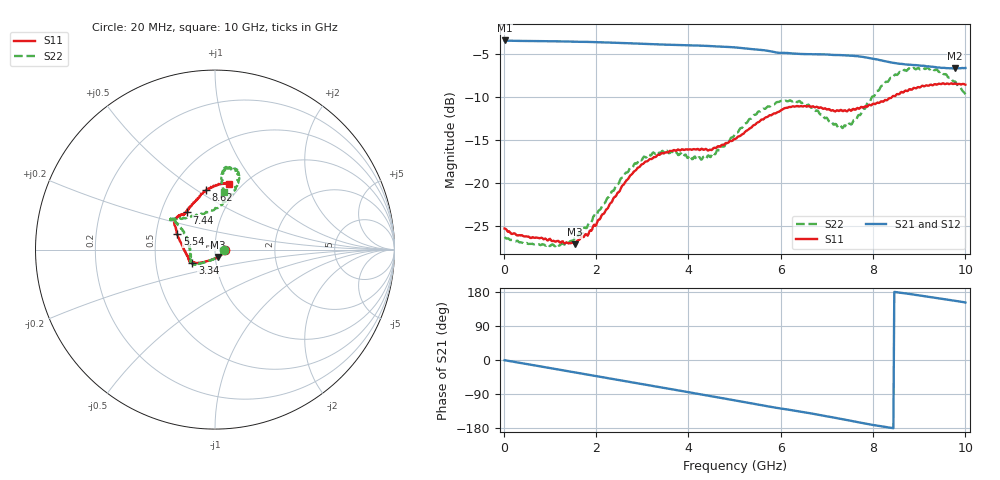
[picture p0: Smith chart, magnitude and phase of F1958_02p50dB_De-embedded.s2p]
! Integrated Device Technology
! Corporate Headquarters
! 6024 Silver Creek Valley Road
! San Jose, CA 95138  USA
! Phone:  1-408-284-8200
! Toll Free:  1-800-223-1366
! Webpage:  http://www.idt.com/
! Timing and RF Division
! 515 Groton Road, Suite 102
! Westford, MA 01886-6024
! Device:  F1958
! Description: 7-bit 0.25 dB Digital Step Attenuator
! Frequency:  0.001 -  6.000 GHz
! Package:  4x4 mm Thin QFN Plastic Package: 24 pin
! Ports:  2 RF, 12 DC
!  Pin  1  = D0
!  Pin  2  = VDD
!  Pin  3  = VMODE
!  Pin  4  = GND
!  Pin  5  = RF1  =  Port 1
!  Pin  6  = GND
!  Pin  7  = GND
!  Pin  8  = GND
!  Pin  9  = GND
!  Pin 10  = GND
!  Pin 11  = GND
!  Pin 12  = GND
!  Pin 13  = GND
!  Pin 14  = RF2  =  Port 2
!  Pin 15  = GND
!  Pin 16  = LE
!  Pin 17  = CLK
!  Pin 18  = DATA
!  Pin 19  = D6
!  Pin 20  = D5
!  Pin 21  = D4
!  Pin 22  = D3
!  Pin 23  = D2
!  Pin 24  = D1
! State:  10
! Atten State:  2.50 dB
! Voltage:  +3.30 Volts
! Current:  0.257 mA
! Data:  The device was measured on a F1958 evaluation board which has
!  individual transmission lines to the RF pins.  Data was collected
!  using a calibrated network analyzer.  The evaluation board was
!  de-embedded using Automatic Fixture Removal (AFR).
!  The reference plane is the edge of the package pin.
! Misc:
!  Action Tracker AT0419
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# GHz S dB R 50
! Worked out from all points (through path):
!   500 points, 20 MHz to 10 GHz, reference 50 ohm
!   highest |S21| = -3.46 dB at 20 MHz (marker M1); lowest = -6.7 dB at 9.78 GHz (marker M2)
!   group delay of S21, straight-line fit = 58.6 ps
!   lowest |S11| = -27.1 dB at 1.54 GHz (marker M3), VSWR 1.09, Z = 51.2 - j4.29 ohm
!   |S11| at or under -10 dB: start of sweep to 8.414 GHz
!   |S22| runs from -27.4 to -6.6 dB; largest |S21 - S12| = 0.0019
!   S11 on the Smith chart (normalised r, x): 20 MHz: 1.11, -0.01; 3.34 GHz: 0.77, -0.12; 5.54 GHz: 0.64, +0.12; 7.44 GHz: 0.67, +0.30; 8.62 GHz: 0.73, +0.55; 10 GHz: 0.88, +0.74
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0.02  -25.32 -2.5  -3.46 -0.6  -3.46 -0.5  -26.30 -2.9
0.96  -26.69 -32.7  -3.54 -20.4  -3.54 -20.3  -27.13 -40.4
1.54  -27.12 -71.5  -3.60 -32.7  -3.60 -32.7  -26.39 -83.2
1.7  -26.27 -83.0  -3.62 -36.0  -3.61 -36.0  -25.82 -95.1
1.86  -25.60 -95.7  -3.63 -39.4  -3.63 -39.4  -24.58 -103.6
2.72  -19.32 -137.8  -3.78 -57.7  -3.77 -57.7  -18.43 -139.2
3.34  -16.73 -149.6  -3.92 -70.9  -3.92 -71.0  -16.35 -148.5
3.36  -16.75 -149.4  -3.93 -71.3  -3.93 -71.4  -16.47 -148.2
4.34  -16.17 -163.8  -4.07 -92.1  -4.09 -92.1  -16.95 -179.2
4.6  -15.95 -169.6  -4.14 -97.7  -4.15 -97.7  -16.47 166.2
5.02  -14.90 174.9  -4.27 -107.0  -4.28 -107.0  -14.22 152.0
5.54  -12.89 157.8  -4.54 -118.2  -4.55 -118.2  -11.70 145.9
6.02  -11.52 148.5  -4.89 -127.9  -4.91 -127.9  -10.49 145.5
6.68  -11.11 137.3  -5.06 -141.4  -5.07 -141.3  -11.26 140.6
7.2  -11.62 130.9  -5.15 -152.9  -5.16 -152.8  -13.19 117.8
7.44  -11.70 127.3  -5.20 -158.5  -5.21 -158.5  -13.50 99.3
7.94  -10.97 116.9  -5.52 -170.2  -5.51 -170.2  -10.49 74.6
8.34  -10.19 106.2  -5.95 -178.2  -5.96 -178.3  -8.13 70.8
8.62  -9.44 98.8  -6.18 177.0  -6.18 177.0  -7.18 73.2
9.28  -8.66 83.2  -6.51 165.1  -6.52 165.1  -6.66 82.4
9.78  -8.45 78.0  -6.71 156.2  -6.73 156.3  -8.24 83.9
10  -8.59 77.5  -6.66 151.6  -6.69 151.7  -9.70 80.7
